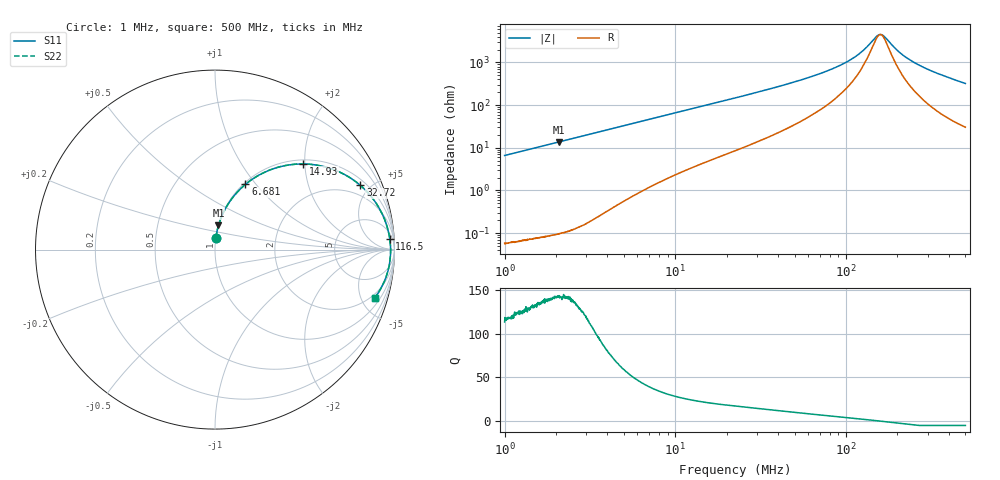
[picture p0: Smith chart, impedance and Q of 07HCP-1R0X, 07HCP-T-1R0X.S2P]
!s-Parameter Generated by FASTRON Sdn. Bhd.
!FASTRON P/N : 07HCP-1R0X, 07HCP/T-1R0X
!Keysight Technologies,E4991B,MY54100416,A.01.15
!Date: Thu Feb 19 15:52:33 2026
!Version  : Rev00 Thu Feb 19 15:52:33 2026
!Data & Calibration Information:
!PortZ  Port1:50+j0  Port2:50+j0
!When reading, reference impedance value at option line is always used.
! Remarks : This data is being provided solely for informational purposes.
!Freq	S11	S21	S12	S22
# Hz S dB R 50
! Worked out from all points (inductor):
!   1601 points, 1 MHz to 500 MHz, reference 50 ohm
!   read as one part in series: L = 1.05 uH near 1.032 MHz
!   highest Q = 143 at 2.084 MHz (marker M1), where L = 1.05 uH
!   self-resonance near 158.7 MHz
!   S11 on the Smith chart (normalised r, x): 1 MHz: 1.00, +0.13; 6.681 MHz: 1.02, +0.88; 14.93 MHz: 1.09, +1.96; 32.72 MHz: 1.32, +4.36; 116.5 MHz: 11, +28; 500 MHz: 1.61, -6.41
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1000000  -23.63 85.7  -0.02 -3.8  -0.02 -3.8  -23.63 85.7
2083607  -17.33 81.8  -0.09 -7.8  -0.09 -7.8  -17.33 81.8
2820919  -14.75 79.0  -0.16 -10.5  -0.16 -10.5  -14.75 79.0
4495866  -10.93 72.6  -0.40 -16.5  -0.40 -16.5  -10.93 72.6
6681481  -7.94 65.0  -0.85 -23.6  -0.85 -23.6  -7.94 65.0
7957584  -6.74 61.0  -1.16 -27.4  -1.16 -27.4  -6.74 61.0
1.115675e7  -4.71 52.3  -2.03 -35.5  -2.03 -35.5  -4.71 52.3
1.492973e7  -3.29 44.2  -3.12 -43.1  -3.12 -43.1  -3.29 44.2
2.236068e7  -1.88 33.2  -5.23 -53.5  -5.23 -53.5  -1.88 33.2
3.271877e7  -1.06 23.9  -7.84 -62.0  -7.84 -62.0  -1.06 23.9
6.307767e7  -0.41 11.6  -13.86 -71.2  -13.86 -71.2  -0.41 11.6
9.01709e7  -0.27 6.6  -18.55 -71.8  -18.55 -71.8  -0.27 6.6
1.165196e8  -0.22 3.5  -23.65 -66.4  -23.65 -66.4  -0.22 3.5
1.284016e8  -0.20 2.4  -26.44 -59.8  -26.44 -59.8  -0.20 2.4
1.488233e8  -0.19 0.7  -31.94 -29.8  -31.94 -29.8  -0.19 0.7
1.553196e8  -0.19 0.2  -33.14 -11.1  -33.14 -11.1  -0.19 0.2
1.646376e8  -0.19 -0.4  -32.89 18.2  -32.89 18.2  -0.19 -0.4
1.77937e8  -0.19 -1.3  -30.10 45.6  -30.10 45.6  -0.19 -1.3
2.110998e8  -0.20 -3.3  -24.19 66.7  -24.19 66.7  -0.20 -3.3
2.59353e8  -0.23 -5.9  -19.56 72.4  -19.56 72.4  -0.23 -5.9
3.484114e8  -0.34 -10.1  -15.01 72.6  -15.01 72.6  -0.34 -10.1
5e8  -0.63 -16.7  -10.79 67.9  -10.79 67.9  -0.63 -16.7
